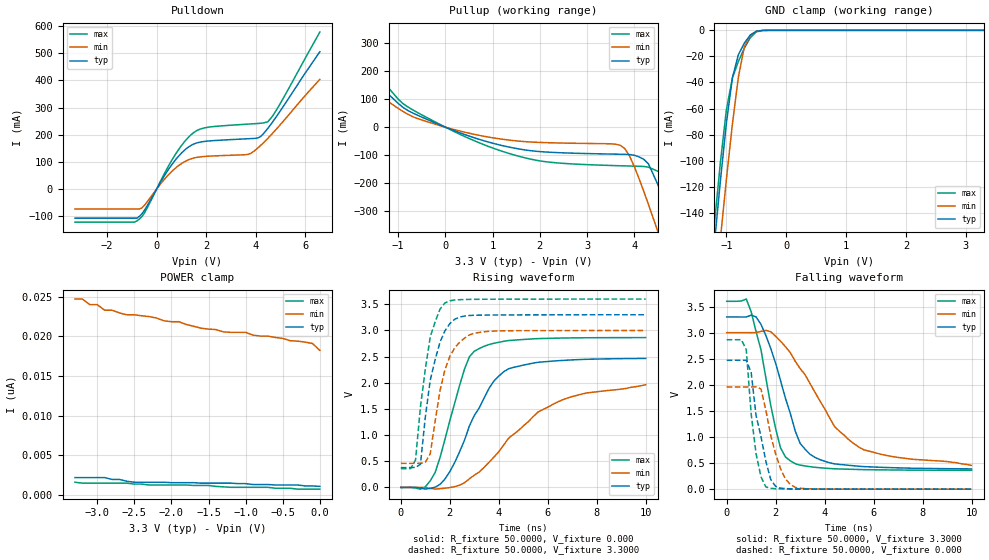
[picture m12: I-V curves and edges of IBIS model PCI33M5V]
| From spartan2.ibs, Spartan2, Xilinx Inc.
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|   Model PCI33M5V
[Model]   PCI33M5V
Model_type   I/O
Polarity   Non-Inverting
Enable   Active-Low
Vinl =   0.800V
Vinh =   2.000V
Vmeas =  1.500V
Cref =  50.00pF
Rref =  1.0M
Vref =   0.0V
C_comp   6.5000pF   5.0000pF   8.0000pF
[Temperature Range]   27.0000   100.0000   0.000
[Voltage Range]   3.3000V   3.0000V   3.6000V
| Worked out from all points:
|   slope of the pulldown table from 0 to 0.495 V, typ, clamps not added: 6.65 ohm
|   slope of the pullup table from 0 to 0.495 V, typ, clamps not added: 15.7 ohm
|   GND clamp passes 1 mA (typ) near -0.51 V on its own axis
|   rising waveform, R_fixture 50.0000, V_fixture 0.000: 20-80 % time 1.5ns typ, 2.72ns min, 1.02ns max; typ from 0 V to 2.46 V
|   rising waveform, R_fixture 50.0000, V_fixture 3.3000: 20-80 % time 649ps typ, 684ps min, 559ps max; typ from 0.379 V to 3.3 V
|   falling waveform, R_fixture 50.0000, V_fixture 3.3000: 20-80 % time 1.14ns typ, 2.2ns min, 844ps max; typ from 3.3 V to 0.388 V
|   falling waveform, R_fixture 50.0000, V_fixture 0.000: 20-80 % time 560ps typ, 625ps min, 386ps max; typ from 2.47 V to 0 V
[Pulldown]
| voltage   I(typ)   I(min)   I(max)
-3.3V     -107.2mA   -73.42mA   -122mA
-800mV    -107.2mA   -73.42mA   -117.5mA
-500mV    -79.21mA   -60.49mA   -89.17mA
700mV     100.3mA    72.17mA    119.1mA
1.1V      140.8mA    99.09mA    171.3mA
1.5V      165.7mA    114.3mA    207.9mA
2.1V      177mA      121mA      227.9mA
3.7V      185.2mA    127.7mA    239.2mA
4.2V      193mA      160mA      242.2mA
4.5V      223.7mA    187mA      247.8mA
4.9V      274.3mA    226.6mA    299.3mA
6.6V      505.5mA    403.9mA    577.9mA
[Pullup]
| voltage   I(typ)   I(min)   I(max)
-3.3V     447.6mA    344.1mA    537.5mA
-2.7V     358.3mA    273.6mA    429.8mA
-2.3V     295.4mA    224.1mA    355.1mA
-600mV    43.62mA    31.46mA    53.31mA
1.6V      -79.23mA   -50.72mA   -106.2mA
3.7V      -97.01mA   -64.82mA   -138.3mA
3.9V      -98.14mA   -103.8mA   -139.2mA
4.2V      -115mA     -229.6mA   -140.8mA
4.5V      -206mA     -374.5mA   -158mA
4.9V      -403.9mA   -575.1mA   -261.6mA
5.1V      -509.1mA   -676.8mA   -357.4mA
6.6V      -1.32A     -1.449A    -1.171A
[GND_clamp]
| voltage   I(typ)   I(min)   I(max)
-3.3V     -1.286A    -1.273A    -1.289A
-1.2V     -163.3mA   -206.7mA   -148.3mA
-1.1V     -115.2mA   -159.6mA   -101mA
-1V       -71.04mA   -114.2mA   -60.78mA
-900mV    -36.42mA   -71.86mA   -36.53mA
-800mV    -18.72mA   -35.86mA   -23.84mA
-700mV    -9.715mA   -12.62mA   -13.63mA
-600mV    -3.608mA   -3.649mA   -5.602mA
-500mV    -692.7uA   -854.2uA   -1.156mA
-400mV    -68.48uA   -138.7uA   -98.54uA
-300mV    -4.365uA   -16.73uA   -4.627uA
3.3V      1.048nA    19.44nA    40.4nA
[POWER_clamp]
| voltage   I(typ)   I(min)   I(max)
-3.3V     2.212nA    24.68nA    1.63nA
-3.2V     2.212nA    24.68nA    1.513nA
-3.1V     2.212nA    23.98nA    1.513nA
-3V       2.212nA    23.98nA    1.513nA
-2.9V     2.212nA    23.28nA    1.513nA
-2.6V     1.746nA    22.7nA     1.513nA
-1.9V     1.572nA    21.83nA    1.281nA
-1.3V     1.513nA    20.55nA    1.048nA
-1V       1.455nA    20.49nA    989.5pA
-900mV    1.339nA    20.14nA    989.5pA
-100mV    1.164nA    19.09nA    756.7pA
0V        1.106nA    18.22nA    756.7pA
[Ramp]
| variable   typ   min   max
dV/dt_r   1.4790/1.4894n   1.1430/2.5760n   1.7178/1.0217n
dV/dt_f   1.7469/1.1800n   1.4917/2.0700n   1.9432/0.7937n
R_load = 50.0000
[Rising Waveform]
R_fixture = 50.0000
V_fixture = 0.000
| time   V(typ)   V(min)   V(max)
0s        0V         0V         0V
800ps     -11.1mV    1.605mV    -33mV
1.4ns     4.272mV    -31.48mV   286.3mV
2ns       301mV      -3.101mV   1.276V
2.6ns     903.2mV    91.09mV    2.261V
3ns       1.375V     234.1mV    2.603V
3.8ns     2.032V     579.2mV    2.754V
4.4ns     2.268V     939.7mV    2.807V
6.6ns     2.426V     1.673V     2.854V
10ns      2.465V     1.961V     2.863V
[Rising Waveform]
R_fixture = 50.0000
V_fixture = 3.3000
V_fixture_min = 3.0000
V_fixture_max = 3.6000
| time   V(typ)   V(min)   V(max)
0s        378.9mV    460.2mV    359.3mV
400ps     379.5mV    460.4mV    361.4mV
600ps     383mV      461mV      525.9mV
800ps     442mV      461.3mV    1.538V
1.2ns     2.049V     641.4mV    2.873V
1.6ns     2.776V     1.852V     3.408V
1.8ns     2.993V     2.248V     3.525V
2.2ns     3.213V     2.666V     3.581V
3ns       3.29V      2.946V     3.594V
10ns      3.299V     2.998V     3.599V
[Falling Waveform]
R_fixture = 50.0000
V_fixture = 3.3000
V_fixture_min = 3.0000
V_fixture_max = 3.6000
| time   V(typ)   V(min)   V(max)
0s        3.3V       3V         3.6V
800ps     3.299V     3V         3.643V
1.4ns     3.159V     3.023V     2.673V
2.2ns     2.081V     2.834V     790.7mV
2.6ns     1.45V      2.615V     542.5mV
3ns       877.6mV    2.312V     460mV
3.4ns     670.4mV    2.027V     431.2mV
4.4ns     485.1mV    1.204V     390.7mV
5.4ns     439.7mV    805.6mV    376.9mV
10ns      388.5mV    456.5mV    361.4mV
[Falling Waveform]
R_fixture = 50.0000
V_fixture = 0.000
| time   V(typ)   V(min)   V(max)
0s        2.47V      1.959V     2.864V
800ps     2.47V      1.959V     2.674V
1ns       2.236V     1.959V     1.441V
1.2ns     1.409V     1.961V     678.9mV
1.4ns     1.012V     1.921V     237.7mV
1.6ns     534.2mV    1.515V     43.64mV
1.8ns     183.3mV    1.025V     15.88mV
2.2ns     20.59mV    390.8mV    6.13mV
2.8ns     4.561mV    35.56mV    2.547mV
10ns      281.4uV    477.3uV    210.6uV
